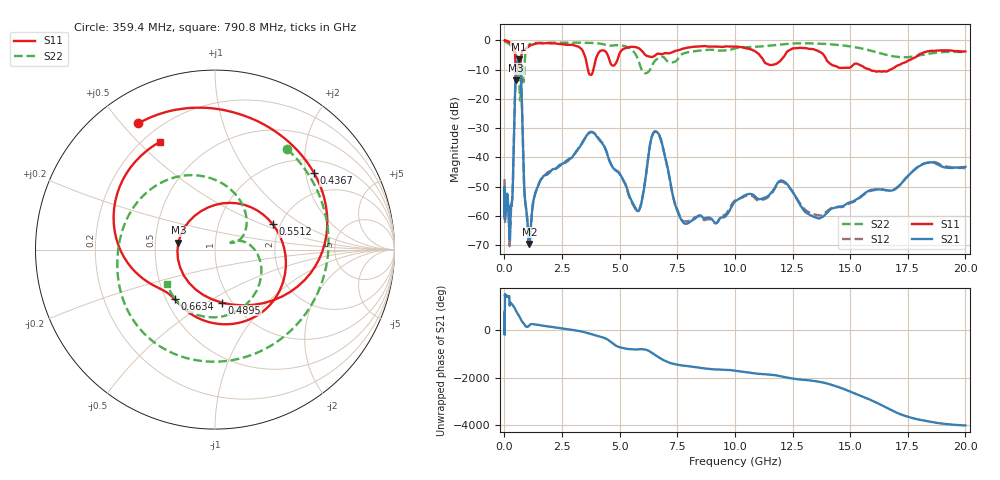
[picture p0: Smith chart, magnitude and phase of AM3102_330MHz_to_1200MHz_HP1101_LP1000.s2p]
! Date/Time: Tue, Sep 11, 2018 5:22 PM
! Network Analyzer: Agilent Technologies E8362B Rev: A.07.50.63
! Sweep from 0.010 to 20.000 GHz, 1601 Points, Sweep Type: LOG
! Power Supply: 4.949 V, 0.001 A
# Hz S DB R 50
!freq MagS11 AngS11 MagS21 AngS21 MagS12 AngS12 MagS22 AngS22
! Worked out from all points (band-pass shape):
!   1601 points, 10 MHz to 20 GHz, reference 50 ohm
!   highest |S21| = -6.45 dB at 632.6 MHz (marker M1); lowest = -69.7 dB at 1.087 GHz (marker M2)
!   |S21| within 3 dB of the highest: 505.9 MHz to 702.3 MHz (196.5 MHz wide, 32.5 % of centre)
!   lowest |S11| = -13.6 dB at 510.8 MHz (marker M3), VSWR 1.52, Z = 33 + j2.6 ohm
!   |S11| at or under -10 dB: 487.6 MHz to 542.3 MHz (54.7 MHz wide, 10.6 % of centre); 3.625 GHz to 3.86 GHz (234.7 MHz wide, 6.27 % of centre); 15.86 GHz to 16.74 GHz (884.9 MHz wide, 5.43 % of centre)
!   |S22| runs from -20.6 to -0.2 dB; largest |S21 - S12| = 0.0078
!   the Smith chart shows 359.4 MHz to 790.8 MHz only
!   S11 on the Smith chart (normalised r, x): 359.4 MHz: 0.13, +0.55; 436.7 MHz: 1.34, +2.23; 489.5 MHz: 0.90, -0.58; 551.2 MHz: 1.83, +0.59; 663.4 MHz: 0.55, -0.35; 790.8 MHz: 0.26, +0.58
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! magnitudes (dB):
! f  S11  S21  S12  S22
! 10 MHz  0.0  -50.3  -47.5  -0.2
! 35.55 MHz  -0.1  -58.8  -57.7  -0.4
! 126.4 MHz  -0.2  -53.4  -54.2  -0.8
! 233.3 MHz  -0.7  -68.3  -69.4  -1.3
! 359.4 MHz  -1.7  -51.2  -51.4  -3.2
! 436.7 MHz  -3.1  -25.8  -25.8  -4.1
! 447.2 MHz  -3.6  -22.6  -22.6  -4.1
! 489.5 MHz  -10.5  -11.8  -11.9  -4.6
! 510.8 MHz  -13.6  -9.0  -9.1  -5.2
! 551.2 MHz  -9.1  -7.4  -7.4  -5.9
! 632.6 MHz  -8.0  -6.4  -6.5  -11.1
! 663.4 MHz  -9.0  -6.8  -6.8  -18.3
! 790.8 MHz  -3.4  -30.6  -30.6  -9.7
! 878 MHz  -3.0  -52.8  -53.1  -8.4
! 1.087 GHz  -1.9  -69.7  -69.1  -1.3
! 1.59 GHz  -1.0  -47.5  -47.4  -0.8
! 3.811 GHz  -11.3  -31.4  -31.3  -0.8
! 5.652 GHz  -2.2  -56.8  -57.3  -4.3
! 6.58 GHz  -4.8  -31.1  -31.3  -6.6
! 7.92 GHz  -2.5  -62.7  -61.9  -4.1
! 13.68 GHz  -3.9  -60.9  -59.8  -1.1
! 20 GHz  -3.8  -43.2  -43.7  -4.0
